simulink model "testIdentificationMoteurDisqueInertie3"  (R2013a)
settings: Solver=ode45  StartTime=0  StopTime=1  FixedStep=1e-3  MaxStep=SimParam.Te  RelTol=1e-4  AbsTol=1e-4
PreLoadFcn:
  | warning('off','sm:sli:setup:compile:LocalSolverNotSupported')
model workspace (MAT data in the model file):
  handle : class17 (value not decoded)
  handle : class17 (value not decoded)
undefined symbols (not defined in the file or in its folder): SimParam

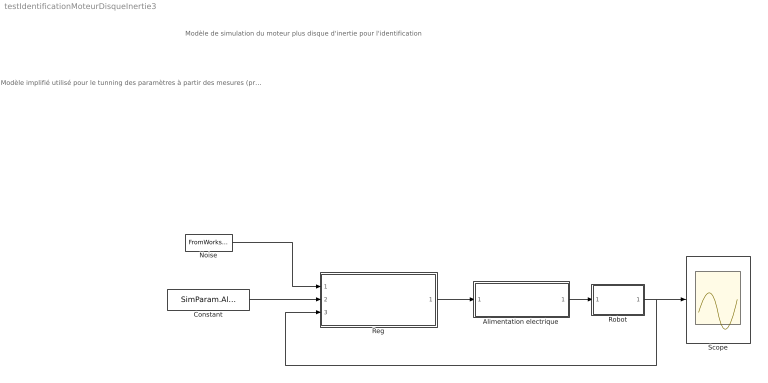
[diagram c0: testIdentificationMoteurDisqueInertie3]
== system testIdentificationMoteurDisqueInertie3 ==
  note: Modèle de simulation du moteur plus disque d'inertie pour l'identification
  note: Modèle implifié utilisé pour le tunning des paramètres à partir des mesures (prbs) effectuée sur le robot (Idem testIdentificationMoteur mais avec un élèment flexible dans le moteur) - Régulateur PID simple avec quantification codeur - Alimentation éléctrique modélisée par une fonction de transfert d'ordre deux avec delais (delais du contrôle) - Méchanique comprennant uniquement un modèle du moteur (inertie + frottement + 1ddl flexible en torsion) + frottement sec - Signaux d'exitation comprennant un bruit blanc et un signal cyclique (PRBS)
  Alimentation electrique : Subsystem
  Constant : Constant  Value=SimParam.Alpha_c
  Noise : FromWorkspace  VariableName=SimIn  SampleTime=SimParam.Te  Interpolate=off  OutputAfterFinalValue=Holding final value
  Reg : Subsystem
  Robot : Subsystem
  Scope : Scope
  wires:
  Noise/1 -> Reg/1(Noise)
  Alimentation electrique/1(Torque_out) -> Robot/1(Tmotor)
  Robot/1(Out1) -> Scope/1, Reg/3(Alpha)
  Reg/1(Torque) -> Alimentation electrique/1(Torque_in)
  Constant/1 -> Reg/2(Alpha_c)

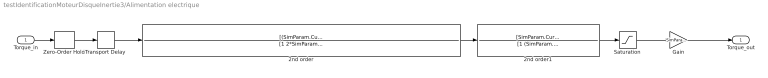
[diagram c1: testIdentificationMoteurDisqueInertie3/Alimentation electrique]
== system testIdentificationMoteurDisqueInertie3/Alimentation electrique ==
  Torque_in : Inport
  2nd order : TransferFcn  Numerator=[(SimParam.CurrentLoop.f0*2*pi)^2]  Denominator=[1 2*SimParam.CurrentLoop.Cr*(SimParam.CurrentLoop.f0*2*pi) (SimParam.CurrentLoop.f0*2*pi)^2]
  2nd order1 : TransferFcn  Numerator=[SimParam.CurrentLoop.f1*2*pi]  Denominator=[1 (SimParam.CurrentLoop.f1*2*pi)]
  Gain : Gain  Gain=SimParam.Grel
  Saturation : Saturate  UpperLimit=10  LowerLimit=-10
  Transport Delay : TransportDelay  DelayTime=SimParam.tauElec
  Zero-Order Hold : ZeroOrderHold  SampleTime=SimParam.TeElec
  Torque_out : Outport
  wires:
  Saturation/1 -> Gain/1
  Torque_in/1 -> Zero-Order Hold/1
  Zero-Order Hold/1 -> Transport Delay/1
  2nd order/1 -> 2nd order1/1
  2nd order1/1 -> Saturation/1
  Gain/1 -> Torque_out/1
  Transport Delay/1 -> 2nd order/1

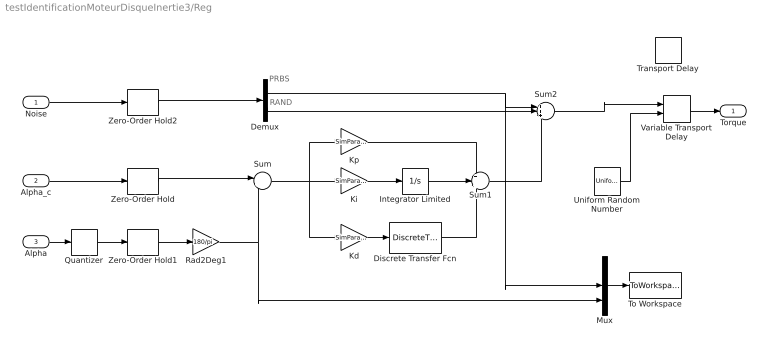
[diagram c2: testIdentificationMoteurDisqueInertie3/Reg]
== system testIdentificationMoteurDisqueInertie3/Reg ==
  note: RAND
  note: PRBS
  Noise : Inport
  Alpha_c : Inport  Port=2
  Alpha : Inport  Port=3
  Demux : Demux  Outputs=2
  Discrete Transfer Fcn : DiscreteTransferFcn  Numerator=[1 0 -1]  Denominator=[2 0 0]
  Integrator Limited : Integrator  LimitOutput=on  UpperSaturationLimit=1  LowerSaturationLimit=-1
  Kd : Gain  Gain=SimParam.Control.Kd/SimParam.Te
  Ki : Gain  Gain=SimParam.Control.Ki*SimParam.Te
  Kp : Gain  Gain=SimParam.Control.Kp
  Mux : Mux  Inputs=3
  Quantizer : Quantizer  QuantizationInterval=SimParam.CoderResol
  Rad2Deg1 : Gain  Gain=180/pi
  Sum : Sum  Inputs=|+-
  Sum1 : Sum  Inputs=+++
  Sum2 : Sum  Inputs=+++
  To Workspace : ToWorkspace  VariableName=simout  SampleTime=SimParam.Te  SaveFormat=Structure With Time
  Transport Delay : TransportDelay  Commented=on  DelayTime=SimParam.tauCtr
  Uniform Random Number : UniformRandomNumber  Minimum=SimParam.tauCtr*0.9  Maximum=SimParam.tauCtr*1.1  SampleTime=SimParam.Te
  Variable Transport Delay : VariableTransportDelay  VariableDelayType=Variable transport delay  MaximumDelay=SimParam.tauCtr*1.2
  Zero-Order Hold : ZeroOrderHold  SampleTime=SimParam.Te
  Zero-Order Hold1 : ZeroOrderHold  SampleTime=SimParam.Te
  Zero-Order Hold2 : ZeroOrderHold  SampleTime=SimParam.Te
  Torque : Outport
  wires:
  Alpha_c/1 -> Zero-Order Hold/1
  Kd/1 -> Discrete Transfer Fcn/1
  Mux/1 -> To Workspace/1
  Zero-Order Hold/1 -> Sum/1
  Alpha/1 -> Quantizer/1
  Quantizer/1 -> Zero-Order Hold1/1
  Noise/1 -> Zero-Order Hold2/1
  Discrete Transfer Fcn/1 -> Sum1/3
  Kp/1 -> Sum1/1
  Sum1/1 -> Sum2/3
  Demux/1 -> Mux/2, Sum2/1
  Ki/1 -> Integrator Limited/1
  Integrator Limited/1 -> Sum1/2
  Sum/1 -> Ki/1, Kp/1, Kd/1
  Zero-Order Hold1/1 -> Rad2Deg1/1
  Rad2Deg1/1 -> Mux/3, Sum/2
  Demux/2 -> Sum2/2
  Zero-Order Hold2/1 -> Demux/1
  Sum2/1 -> Variable Transport Delay/1
  Variable Transport Delay/1 -> Torque/1
  Uniform Random Number/1 -> Variable Transport Delay/2

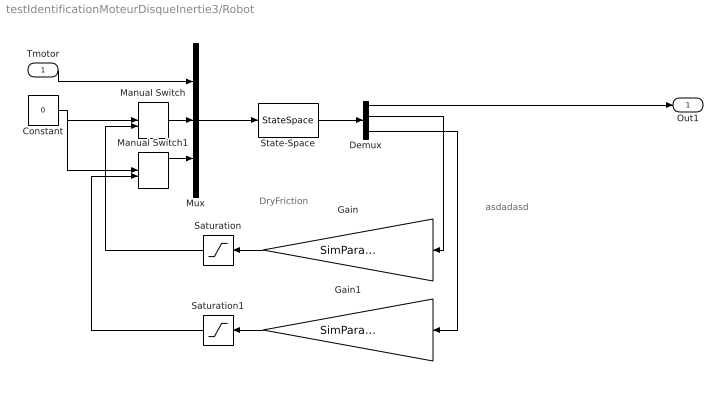
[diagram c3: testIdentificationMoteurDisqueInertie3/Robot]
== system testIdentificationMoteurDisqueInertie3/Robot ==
  note: asdadasd
  note: DryFriction
  Tmotor : Inport
  Constant : Constant  Value=0
  Demux : Demux
  Gain : Gain  Gain=SimParam.CdmotorSlope
  Gain1 : Gain  Gain=SimParam.CdmotorSlope
  Manual Switch : ManualSwitch
  Manual Switch1 : ManualSwitch
  Mux : Mux  Inputs=3
  Saturation : Saturate  UpperLimit=1  LowerLimit=-1
  Saturation1 : Saturate  UpperLimit=1  LowerLimit=-1
  State-Space : StateSpace  A=SimParam.Mec.A  B=SimParam.Mec.B  C=SimParam.Mec.C  D=SimParam.Mec.D
  Out1 : Outport
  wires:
  Gain/1 -> Saturation/1
  Saturation/1 -> Manual Switch/2
  Constant/1 -> Manual Switch/1, Manual Switch1/1
  State-Space/1 -> Demux/1
  Mux/1 -> State-Space/1
  Manual Switch/1 -> Mux/2
  Manual Switch1/1 -> Mux/3
  Demux/2 -> Gain/1
  Gain1/1 -> Saturation1/1
  Saturation1/1 -> Manual Switch1/2
  Demux/4 -> Gain1/1
  Tmotor/1 -> Mux/1
  Demux/1 -> Out1/1
